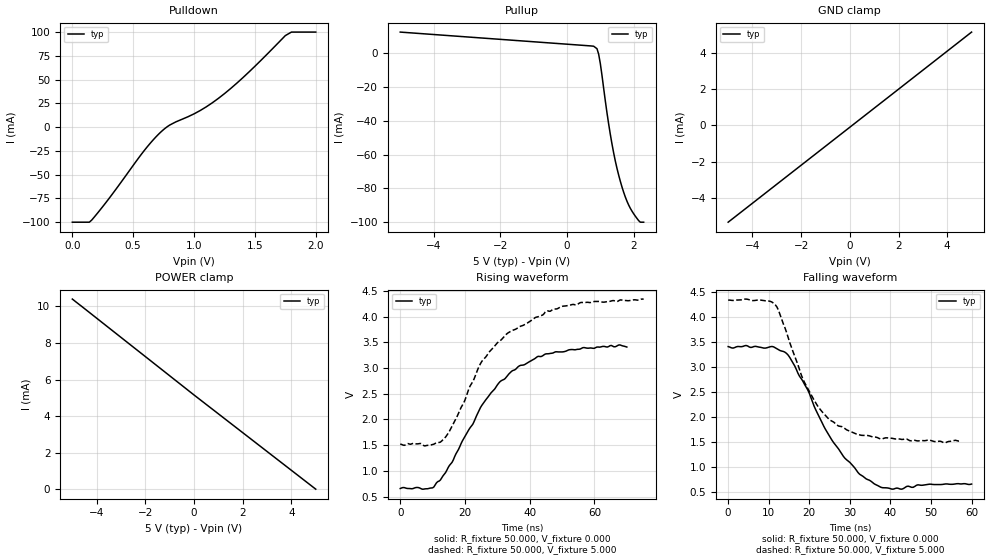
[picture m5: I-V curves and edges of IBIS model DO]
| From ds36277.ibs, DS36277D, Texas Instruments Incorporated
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|   Model DO
[Model]   DO
Model_type   I/O
Vinl = -7
Vinh = 12
Vmeas = 2.5
Vref = 2.5
Cref = 15pF
Rref = 50
|   typ   min   max
|   (nom PVT)   (fast PVT)   (slow PVT)
C_comp   16.737pF   NA   NA
[Voltage Range]   5   NA   NA
[Temperature Range]   27   NA   NA
[Power Clamp Reference]   5   NA   NA
[GND Clamp Reference]   0   0   0
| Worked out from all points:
|   slope of the pulldown table from 0 to 0.75 V, typ, clamps not added: 7.7 ohm
|   slope of the pullup table from 0 to 0.75 V, typ, clamps not added: 682 ohm
|   GND clamp passes 1 mA (typ) near -0.86 V on its own axis
|   falling waveform, R_fixture 50.000, V_fixture 0.000: 20-80 % time 11.1ns typ, NA min, NA max; typ from 3.41 V to 0.658 V
|   falling waveform, R_fixture 50.000, V_fixture 5.000: 20-80 % time 9.35ns typ, NA min, NA max; typ from 4.34 V to 1.52 V
|   rising waveform, R_fixture 50.000, V_fixture 0.000: 20-80 % time 16.8ns typ, NA min, NA max; typ from 0.658 V to 3.41 V
|   rising waveform, R_fixture 50.000, V_fixture 5.000: 20-80 % time 18.4ns typ, NA min, NA max; typ from 1.52 V to 4.34 V
[GND Clamp]
|   Voltage   I(typ)   I(min)  I(max)
-5V       -5.339mA   NA         NA
2V        2.003mA    NA         NA
2.2V      2.214mA    NA         NA
5V        5.154mA    NA         NA
[POWER Clamp]
|   Voltage   I(typ)   I(min)  I(max)
-5V       10.4mA     NA         NA
-4.6V     9.986mA    NA         NA
0V        5.154mA    NA         NA
5V        0A         NA         NA
[Pulldown]
|   Voltage   I(typ)   I(min)   I(max)
0V        -100mA     NA         NA
140mV     -100mA     NA         NA
160mV     -97.7mA    NA         NA
300mV     -75.33mA   NA         NA
600mV     -23.17mA   NA         NA
760mV     -1.477mA   NA         NA
1.05V     17.43mA    NA         NA
1.2V      30.25mA    NA         NA
1.45V     57.86mA    NA         NA
1.75V     96.28mA    NA         NA
1.8V      100mA      NA         NA
2V        100mA      NA         NA
[Pullup]
|   Voltage   I(typ)   I(min)   I(max)
-5V       12.4mA     NA         NA
700mV     4.239mA    NA         NA
900mV     2.581mA    NA         NA
1V        -6.18mA    NA         NA
1.2V      -35.33mA   NA         NA
1.3V      -48.06mA   NA         NA
1.4V      -59.02mA   NA         NA
1.55V     -72.13mA   NA         NA
1.75V     -85.1mA    NA         NA
1.9V      -91.78mA   NA         NA
2.15V     -99.08mA   NA         NA
2.3V      -100mA     NA         NA
[Ramp]
R_load = 50
|   typ   min   max
dV/dt_r   1.728/17.3e-9   NA   NA
dV/dt_f   1.914/9.082e-9   NA   NA
[Falling Waveform]
R_fixture = 50.000
V_fixture = 0.000
C_fixture = 0.000
|  time   V(typ)   V(min)   V(max)
0s        3.409V     NA         NA
10.8ns    3.412V     NA         NA
14.4ns    3.272V     NA         NA
19.6ns    2.545V     NA         NA
21.6ns    2.142V     NA         NA
25.6ns    1.534V     NA         NA
32.4ns    854.6mV    NA         NA
36ns      663mV      NA         NA
40.4ns    555.8mV    NA         NA
60ns      658mV      NA         NA
[Falling Waveform]
R_fixture = 50.000
V_fixture = 5.000
C_fixture = 0.000
|  time   V(typ)   V(min)   V(max)
0s        4.339V     NA         NA
8ns       4.339V     NA         NA
11.6ns    4.247V     NA         NA
12.4ns    4.137V     NA         NA
19.2ns    2.632V     NA         NA
22.8ns    2.14V      NA         NA
27.2ns    1.82V      NA         NA
31.6ns    1.66V      NA         NA
37.6ns    1.56V      NA         NA
57.2ns    1.52V      NA         NA
[Rising Waveform]
R_fixture = 50.000
V_fixture = 0.000
C_fixture = 0.000
|  time   V(typ)   V(min)   V(max)
0s        658mV      NA         NA
10.4ns    688.9mV    NA         NA
16ns      1.166V     NA         NA
26ns      2.347V     NA         NA
30.8ns    2.733V     NA         NA
36.8ns    3.043V     NA         NA
42.4ns    3.223V     NA         NA
48ns      3.316V     NA         NA
67.6ns    3.45V      NA         NA
70ns      3.409V     NA         NA
[Rising Waveform]
R_fixture = 50.000
V_fixture = 5.000
C_fixture = 0.000
|  time   V(typ)   V(min)   V(max)
0s        1.52V      NA         NA
7.6ns     1.486V     NA         NA
13.6ns    1.63V      NA         NA
17.6ns    2.064V     NA         NA
25.2ns    3.129V     NA         NA
33.6ns    3.696V     NA         NA
45.2ns    4.113V     NA         NA
50ns      4.199V     NA         NA
56ns      4.276V     NA         NA
75.2ns    4.339V     NA         NA
